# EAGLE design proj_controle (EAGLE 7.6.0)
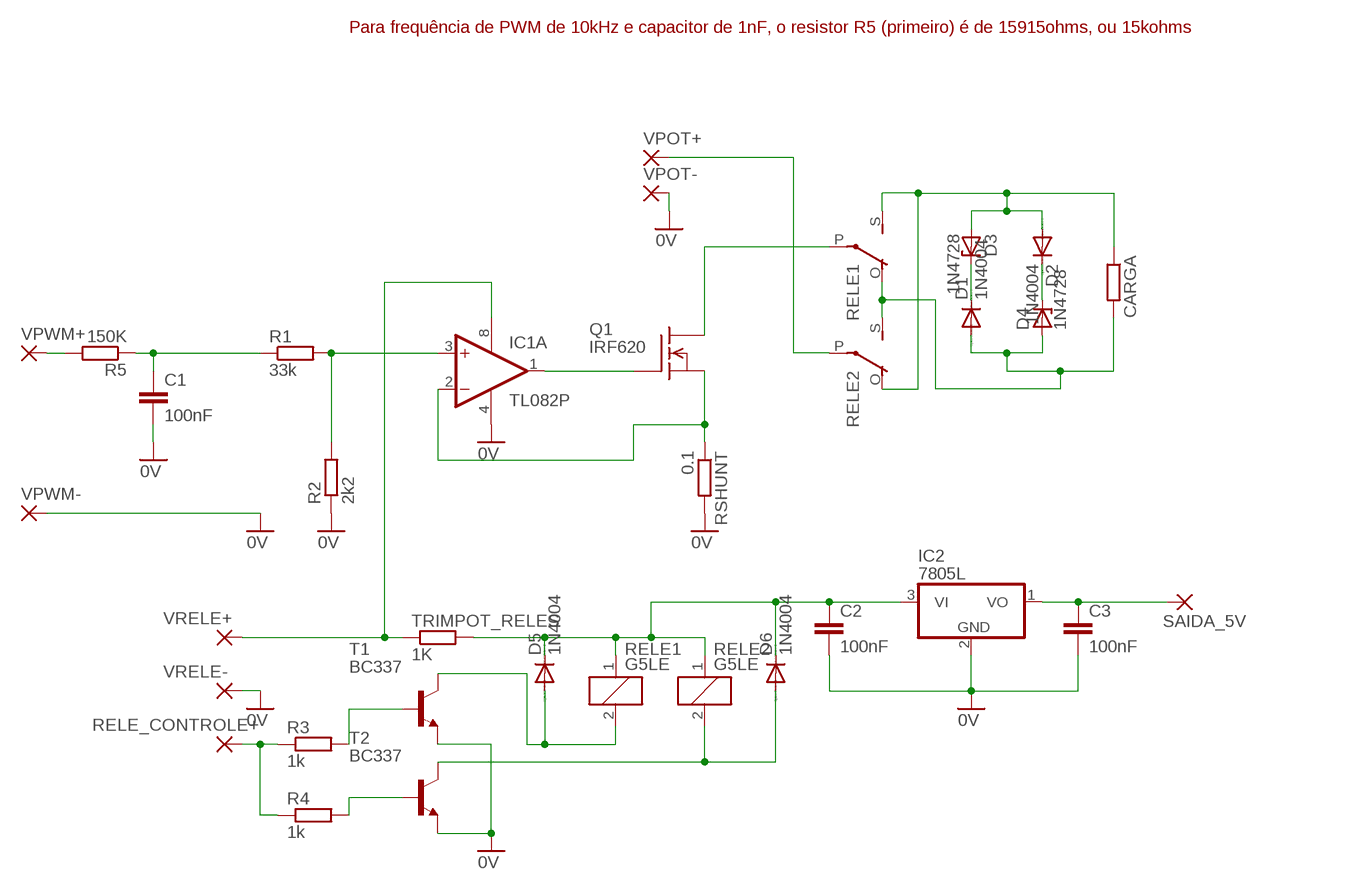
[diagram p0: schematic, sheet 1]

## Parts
C1  100nF  C-EU050-025X075  [C050-025X075]
C2  100nF  C-EU050-025X075  [C050-025X075]
C3  100nF  C-EU050-025X075  [C050-025X075]
CARGA  R-EU_0207/10  [0207/10]
D1  1N4004  [DO41-10]
D2  1N4004  [DO41-10]
D3  1N4728  [DO41Z10]
D4  1N4728  [DO41Z10]
D5  1N4004  [DO41-10]
D6  1N4004  [DO41-10]
IC1  TL082P  [DIL08]
IC2  7805L  [TO92]
Q1  IRF620  [TO220]
R1  33k  R-EU_0207/10  [0207/10]
R2  2k2  R-EU_0207/10  [0207/10]
R3  1k  R-EU_0207/10  [0207/10]
R4  1k  R-EU_0207/10  [0207/10]
R5  150K  R-EU_0207/10  [0207/10]
RELE1  G5LE  [G5LE]
RELE2  G5LE  [G5LE]
RELE_CONTROLE+  3,17/1,1  [3,17/1,1]
RSHUNT  0.1  R-EU_0617/22  [0617/22]
SAIDA_5V  3,17/1,1  [3,17/1,1]
T1  BC337  [TO92]
T2  BC337  [TO92]
TRIMPOT_RELES  1K  R-EU_0207/10  [0207/10]
VPOT+  3,17/1,1  [3,17/1,1]
VPOT-  3,17/1,1  [3,17/1,1]
VPWM+  3,17/1,1  [3,17/1,1]
VPWM-  3,17/1,1  [3,17/1,1]
VRELE+  3,17/1,1  [3,17/1,1]
VRELE-  3,17/1,1  [3,17/1,1]

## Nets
0V: C1.2 C2.2 C3.2 IC1.4(P:V-) IC2.2(GND) R2.1 RSHUNT.2 T1.1(E) T2.1(E) VPOT-.1(P) VPWM-.1(P) VRELE-.1(P)
N$1: D1.C D3.C
N$2: IC1.3(A:+IN) R1.2 R2.2
N$3: IC1.1(A:OUT) Q1.1(G)
N$4: IC1.2(A:-IN) Q1.3(S) RSHUNT.1
N$5: C1.1 R1.1 R5.1
N$6: R5.2 VPWM+.1(P)
N$7: D2.C D4.C
N$8: Q1.2(D) RELE1.P(2:P)
N$10: RELE2.P(2:P) VPOT+.1(P)
N$11: CARGA.1 D2.A D3.A RELE1.S(2:S) RELE2.O(2:O)
N$12: D6.A RELE2.2 T2.3(C)
N$13: D5.A RELE1.2 T1.3(C)
N$14: R3.1 R4.1 RELE_CONTROLE+.1(P)
N$15: R3.2 T1.2(B)
N$16: C2.1 D5.C D6.C IC2.3(VI) RELE1.1 RELE2.1 TRIMPOT_RELES.2
N$17: R4.2 T2.2(B)
N$18: CARGA.2 D1.A D4.A RELE1.O(2:O) RELE2.S(2:S)
N$19: C3.1 IC2.1(VO) SAIDA_5V.1(P)
N$20: IC1.8(P:V+) TRIMPOT_RELES.1 VRELE+.1(P)
Unconnected: IC1.5(B:+IN) IC1.6(B:-IN) IC1.7(B:OUT)

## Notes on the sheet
- Para frequência de PWM de 10kHz e capacitor de 1nF, o resistor R5 (primeiro) é de 15915ohms, ou 15kohms

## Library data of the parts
C1-C3 = rcl:C-EU: CAPACITOR, European symbol
CARGA R1-R5 TRIMPOT_RELES = rcl:R-EU_: RESISTOR, European symbol
D1 D2 D5 D6 = diode:1N4004: DIODE
D3 D4 = diode:1N4728: Z DIODE
IC1 = linear:TL082: OP AMP Data sheet; DATA_SHEET: <a href="http://www.ti.com/lit/ds/symlink/tl084a.pdf"> Data sheet </a>
IC2 = linear:78*: Positive VOLTAGE REGULATOR Source: http://cache.national.com/ds/LM/LM78L05.pdf http://www.fairchildsemi.com/ds/LM/LM7805.pdf
Q1 = transistor-fet:IRF620: N-Channel Enhancement MOSFET (HEXFET); 200V; 5,2A; 0,8Ohm
RELE1 RELE2 = relay:G5LE: RELAY 1 x switch, 10 A/120 V AC, 8 A/30 V DC, Omron; OC_FARNELL: unknown; OC_NEWARK: unknown
RELE_CONTROLE+ SAIDA_5V VPOT+ VPOT- VPWM+ VPWM- VRELE+ VRELE- = wirepad:3,17/1,1: THROUGH-HOLE PAD
RSHUNT = resistor:R-EU_: RESISTOR, European symbol
T1 T2 = transistor:BC337: NPN TRANSISTOR

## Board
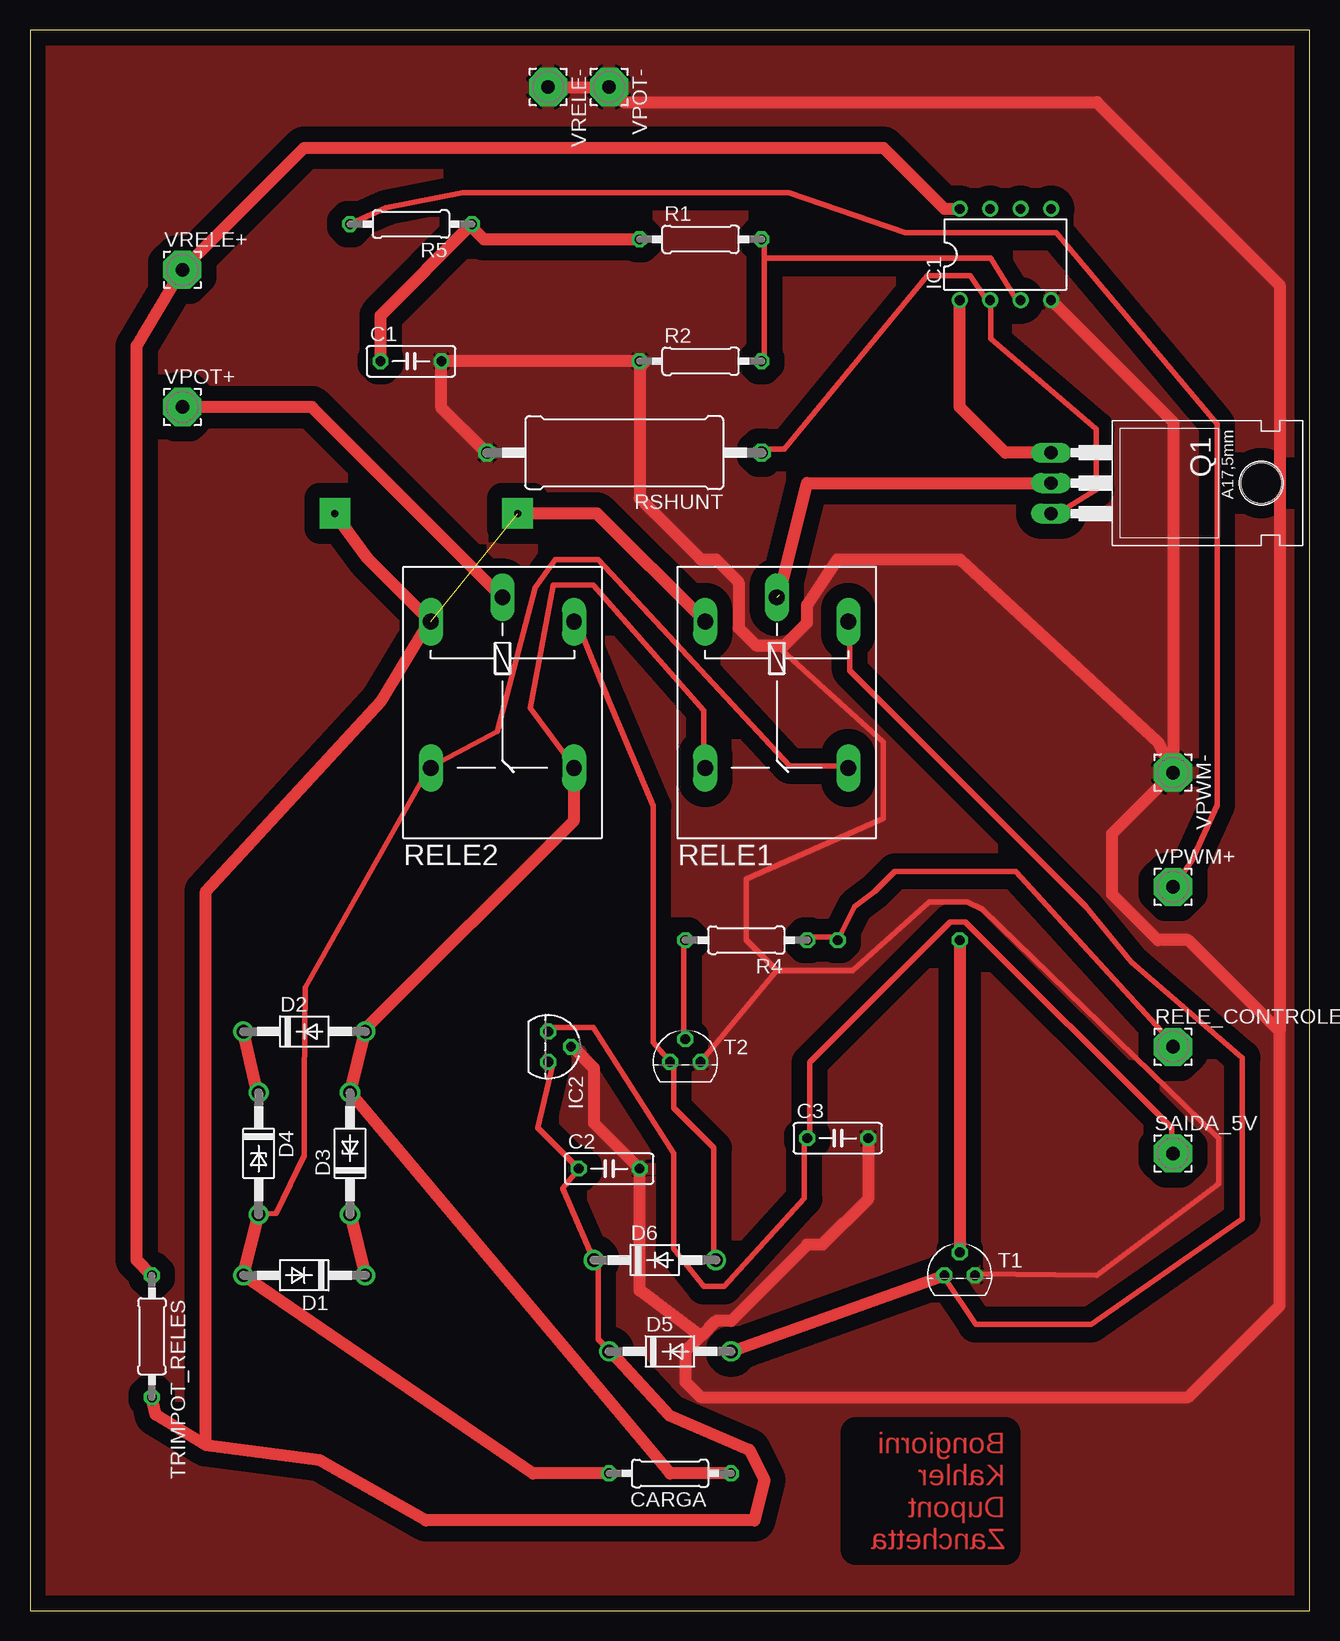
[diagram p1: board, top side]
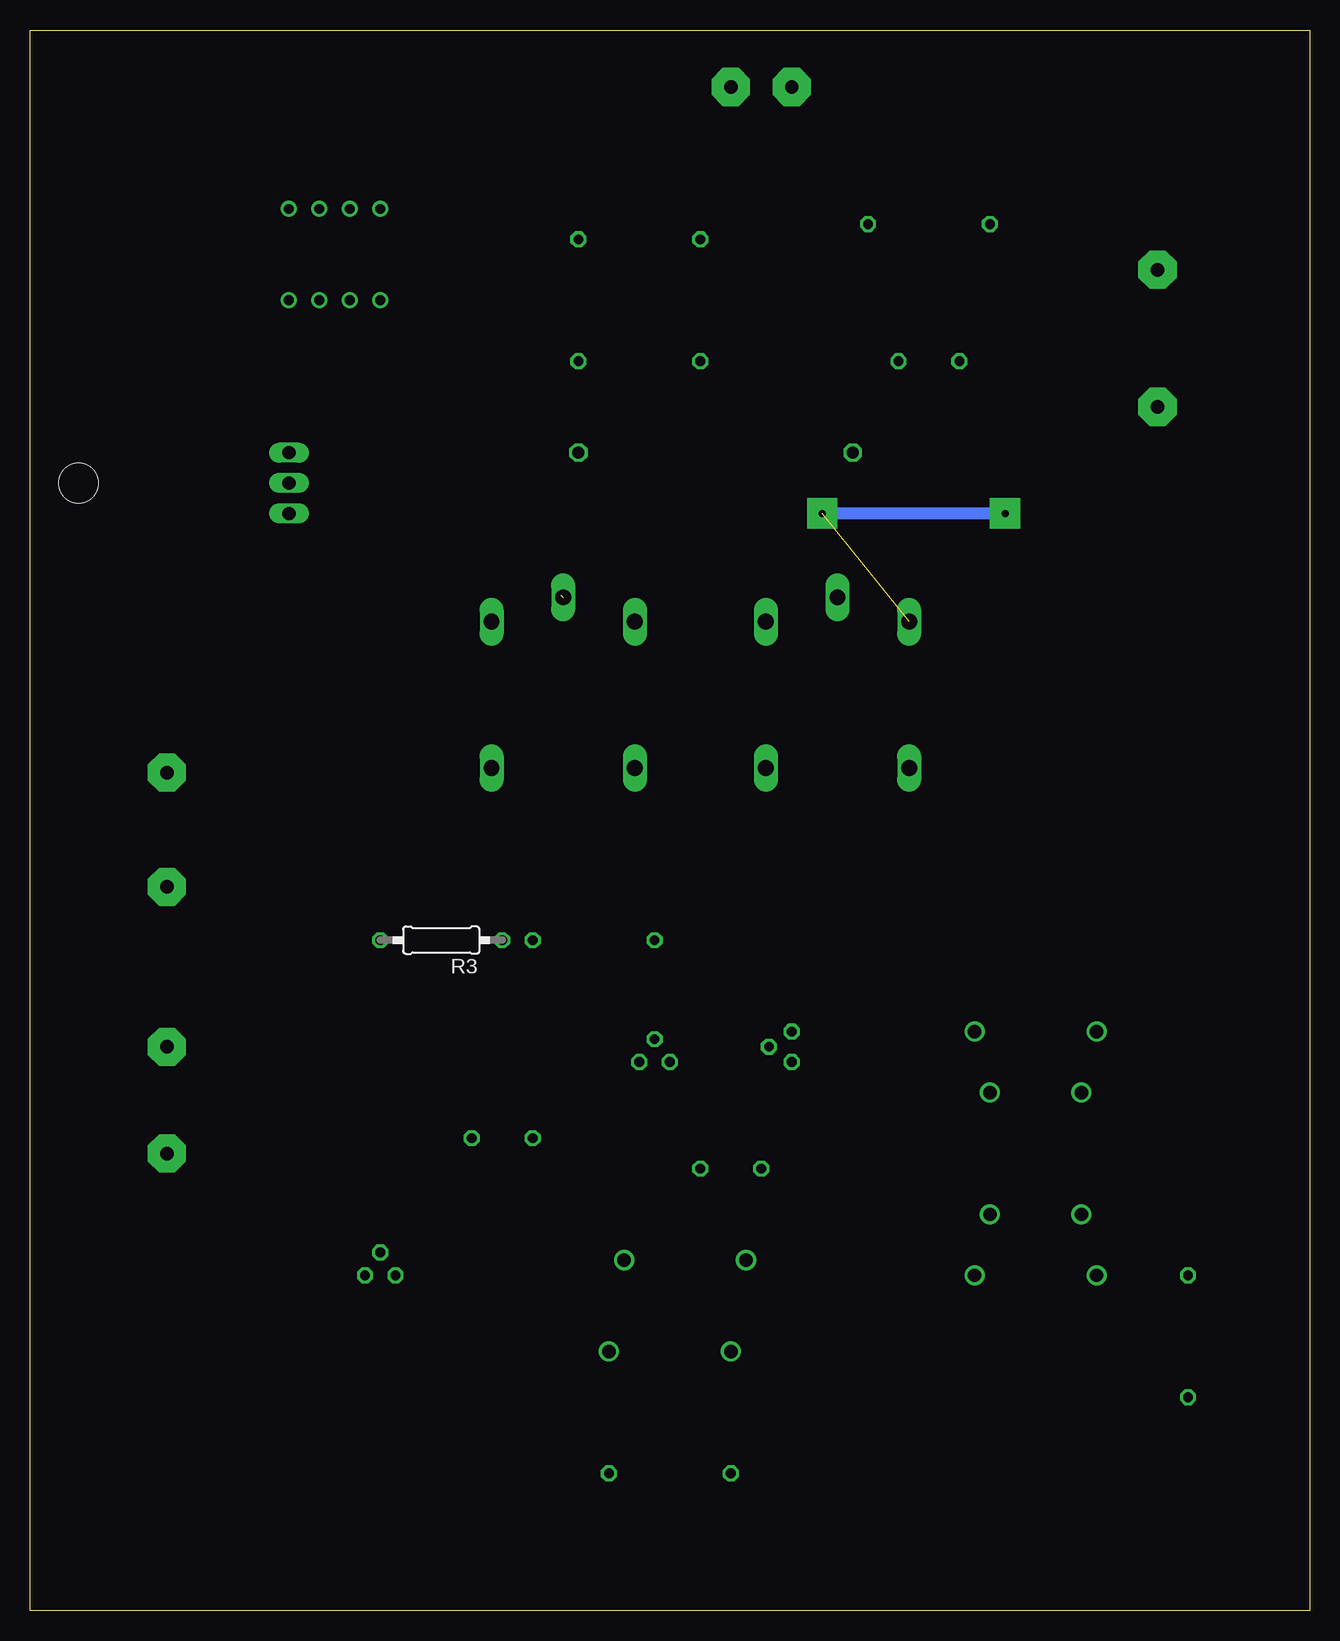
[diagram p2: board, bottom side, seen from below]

Size 106.66 x 131.75 mm. Coordinates in mm from the lower left corner, seen from the top.
Outline: 0,0 106.66,0 106.66,131.75 0,131.75 0,0
Copper layers (1*16): Top 0.035mm / dielectric 1.5mm / Bottom 0.035mm
Design rules "default *": minimum track width 18mil, minimum drill 24mil, track to track 15mil, track to pad 18mil, pad to pad 15mil, via to via 15mil, smd to smd 8mil, copper to edge 40mil, drill to drill 8mil, minimum pad ring 10mil, minimum via ring 8mil, stop-mask expansion 4mil, vias tented up to drill 0mil, thermal gap 10mil

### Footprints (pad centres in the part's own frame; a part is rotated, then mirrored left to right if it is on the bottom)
C050-025X075 = drill 0.813 octagon: 1 -2.54,0; 2 2.54,0
0207/10 = drill 0.813 octagon: 1 -5.08,0; 2 5.08,0
DO41-10 = drill 1.118: A 5.08,0; C -5.08,0
DO41Z10 = drill 1.118: A 5.08,0; C -5.08,0
DIL08 = drill 0.813 pad 1.27: 1 -3.81,-3.81; 2 -1.27,-3.81; 3 1.27,-3.81; 4 3.81,-3.81; 5 3.81,3.81; 6 1.27,3.81; 7 -1.27,3.81; 8 -3.81,3.81
TO92 = drill 0.813 octagon: 1 -1.27,0; 2 0,1.905; 3 1.27,0
TO220 = drill 1.118 long: 1 -2.54,-6.35; 2 0,-6.35; 3 2.54,-6.35 | hole 3.302: 0,11.176
G5LE = drill 1.321 long: 1 -7.493,-5.969; 2 -7.493,5.969; O 4.699,5.969; P -9.525,0; S 4.699,-5.969
3,17/1,1 = drill 1.118 pad 3.175 octagon: 1 0,0
0617/22 = drill 1.016 octagon: 1 -11.43,0; 2 11.43,0
TO92' = drill 0.813 octagon: 1 1.27,0; 2 0,1.905; 3 -1.27,0

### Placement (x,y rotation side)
C1  31.75,104.14 0 top
C2  48.26,36.83 0 top
C3  67.31,39.37 0 top
CARGA  53.34,11.43 180 top
D1  22.86,27.94 180 top
D2  22.86,48.26 0 top
D3  26.67,38.1 90 top
D4  19.05,38.1 270 top
D5  53.34,21.59 0 top
D6  52.07,29.21 0 top
IC1  81.28,113.03 0 top
IC2  43.18,46.99 270 top
Q1  91.44,93.98 270 top
R1  55.88,114.3 0 top
R2  55.88,104.14 0 top
R3  72.39,55.88 180 bottom
R4  59.69,55.88 180 top
R5  31.75,115.57 180 top
RELE1  62.23,74.93 270 top
RELE2  39.37,74.93 270 top
RELE_CONTROLE+  95.25,46.99 0 top
RSHUNT  49.53,96.52 180 top
SAIDA_5V  95.25,38.1 0 top
T1  BC337  [TO92']  77.47,27.94 0 top
T2  BC337  [TO92']  54.61,45.72 0 top
TRIMPOT_RELES  10.16,22.86 270 top
VPOT+  12.7,100.33 0 top
VPOT-  48.26,127 270 top
VPWM+  95.25,60.32 0 top
VPWM-  95.25,69.85 270 top
VRELE+  12.7,111.76 0 top
VRELE-  43.18,127 270 top

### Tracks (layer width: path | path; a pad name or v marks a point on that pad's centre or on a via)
0V
  Top 0.457: 34.37,103.92 C1.2 34.37,104.34 | 37.72,96.8 RSHUNT.2 | 50.71,104.34 R2.1 51.13,103.92 | T1.1 78.79,28.07 88.9,27.94 99.06,35.56 99.06,39.37 79.38,58.42 78.11,59.05 74.93,59.05 68.58,53.34 62.23,53.34 | 45.26,46.93 IC2.2 | 43.59,126.98 VRELE-.1 | 48.2,126.98 VPOT-.1 | 85.5,108.95 IC1.4 | 62.23,53.34 59.69,55.88 59.69,60.96 71.12,66.04 71.12,72.39 62.23,80.45 | T2.1 62.23,53.34
  Top 1: 43.59,126.98 48.2,126.98 | 48.2,126.98 48.26,126.98 VPOT-.1 | VPWM-.1 93.98,72.39 77.47,87.63 67.31,87.63 64.77,83.82 64.77,82.36 62.87,80.45 62.23,80.45 60.52,80.45 59.05,81.92 59.05,85.73 57.15,87.63 55.88,87.63 50.8,92.71 50.8,103.59 51.13,103.92 | IC1.4 95.25,99.06 VPWM-.1 | 45.26,46.93 46.99,45.2 46.99,40.64 C2.2 50.8,26.67 55.88,22.86 | C3.2 69.85,34.29 66.04,30.48 64.77,30.48 58.42,24.13 57.15,24.13 55.88,22.86 | 55.88,22.86 54.61,21.59 54.61,19.05 55.88,17.78 96.52,17.78 104.14,25.4 104.14,48.26 | 104.14,48.26 96.52,55.88 93.98,55.88 90.17,59.69 90.17,64.77 VPWM-.1 | 48.2,126.98 49.44,125.73 88.9,125.73 104.14,110.49 104.14,48.26 | 50.71,104.34 50.51,104.14 C1.2 34.29,100.23 37.72,96.8
  pour Top (isolate 1.27): 0,130.81 106.68,130.81 106.68,0 0,0
N$1
  Top 1: D3.C D1.C
N$2
  Top 0.457: 61.19,112.74 61.19,113.98 R1.2 | 61.19,112.74 61.19,104.34 R2.2 | 61.19,112.74 80.05,112.74 82.14,109.37 IC1.3
N$3
  Top 0.457: 77.53,108.95 IC1.1 | 85.08,96.8 Q1.1
  Top 1: 85.08,96.8 84.8,96.52 81.28,96.52 77.47,100.33 IC1.1
N$4
  Top 0.457: Q1.3 85.5,91.35 88.86,93.45 88.86,98.49 80.05,106.03 80.05,108.95 IC1.2 79.63,109.37 78.37,111.27 74.79,111.27 62.87,96.8 61.19,96.8 RSHUNT.1
N$5
  Top 0.457: 29.34,104.34 C1.1 | 36.46,115.24 R5.1 36.88,115.24 | 50.71,114.4 R1.1
  Top 1: 29.34,104.34 29.21,104.47 29.21,107.95 R5.1 | 36.88,115.24 37.82,114.3 R1.1
N$6
  Top 0.457: R5.2 26.82,115.66 29.7,116.93 36.04,118.19 63.23,118.19 72.92,114.85 85.51,114.85 98.92,98.9 98.92,67.13 96.83,62.5 VPWM+.1
N$7
  Top 0.457: 18.02,48.18 D2.C | 18.85,43.57 D4.C
  Top 1: 18.85,43.57 D2.C
N$8  (1 unrouted)
  Top 1: 62.45,84.65 64.77,93.98 Q1.2
N$9  (via drill 0.6 pad 2.54)
  Bottom 1: v25.4,91.44 v40.64,91.44
N$10
  Top 1: RELE2.P 23.5,100.33 VPOT+.1
N$11
  Top 0.457: 26.84,43.15 D3.A | 45.26,69.98 RELE2.O 45.26,70.4 41.68,75.25 43.59,85.5 44.84,85.48 46.95,85.48 56.16,75.01 56.16,70.4 RELE1.S | 28.08,48.6 D2.A
  Top 1: D2.A D3.A 53.34,11.43 CARGA.1 | 28.08,48.6 45.34,65.86 RELE2.O
N$12
  Top 0.457: D6.A 57,29.32 57,38.54 53.65,41.9 53.65,45.67 T2.3 51.96,47.36 51.96,67.06 48.22,75.87 45.68,82.13 RELE2.2
N$13
  Top 0.457: RELE1.2 68.31,82.13 68.31,78.36 87.97,58.7 91.78,54.05 101.03,46.08 101.03,32.64 88.43,23.85 78.8,23.85 76.28,27.65 T1.3
  Top 1: D5.A T1.3
N$14
  Top 0.457: R4.1 64.96,56.15 67.06,56.15 R3.1 68.75,58.69 70.41,59.96 72.07,61.62 82.13,61.62 95.14,47.35 RELE_CONTROLE+.1
N$15
  Top 0.457: 77.53,30.16 T1.2 | 77.53,55.73 R3.2
  Top 1: 77.53,55.73 77.47,55.66 T1.2
N$16  (1 unrouted)
  Top 0.457: IC2.3 43.59,45.67 42.32,40.22 45.67,36.87 C2.1 44.4,35.18 46.94,29.32 D6.C 47.36,28.91 47.36,22.62 48.2,21.78 D5.C 48.62,21.36 | 33.11,82.13 RELE2.1
  Top 1: 14.66,13.78 24.21,12.51 33.02,7.51 60.36,7.51 61.2,10.88 59.93,13.41 53.25,16.28 48.62,21.36 | 14.66,13.78 10.46,16.32 TRIMPOT_RELES.2 | 33.11,82.13 29.3,75.87 14.66,59.96 14.66,13.78 | RELE2.1 28.19,87.63 25.4,91.44 | RELE1.1 47.24,91.44 40.64,91.44
N$17
  Top 0.457: T2.2 54.48,47.76 54.48,55.73 R4.2
N$18
  Top 0.457: D4.A 20.54,33.1 22.85,37.95 22.85,44.2 22.95,51.92 33.11,69.98 RELE2.S 33.53,70.4 38.94,73.27 42.11,85.28 43.79,87.59 47.37,87.59 63.3,70.4 67.89,70.4 RELE1.O
  Top 1: CARGA.2 41.91,11.43 D1.A D4.A
N$19
  Top 0.457: IC2.1 43.59,48.6 46.95,48.6 53.65,38.1 53.65,30.16 56.16,27.01 57.84,27.01 64.54,34.35 64.54,38.96 C3.1 64.96,39.38 64.96,45.67 76.69,57.4 77.95,57.4 95.14,40.22 95.14,38.12 SAIDA_5V.1
N$20
  Top 0.457: 12.57,111.47 VRELE+.1
  Top 1: IC1.8 76.2,116.84 71.12,121.92 22.86,121.92 VRELE+.1 8.89,105.41 8.89,29.21 TRIMPOT_RELES.1

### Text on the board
Top: Bongiorni / Kahler / Dupont / Zanchetta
